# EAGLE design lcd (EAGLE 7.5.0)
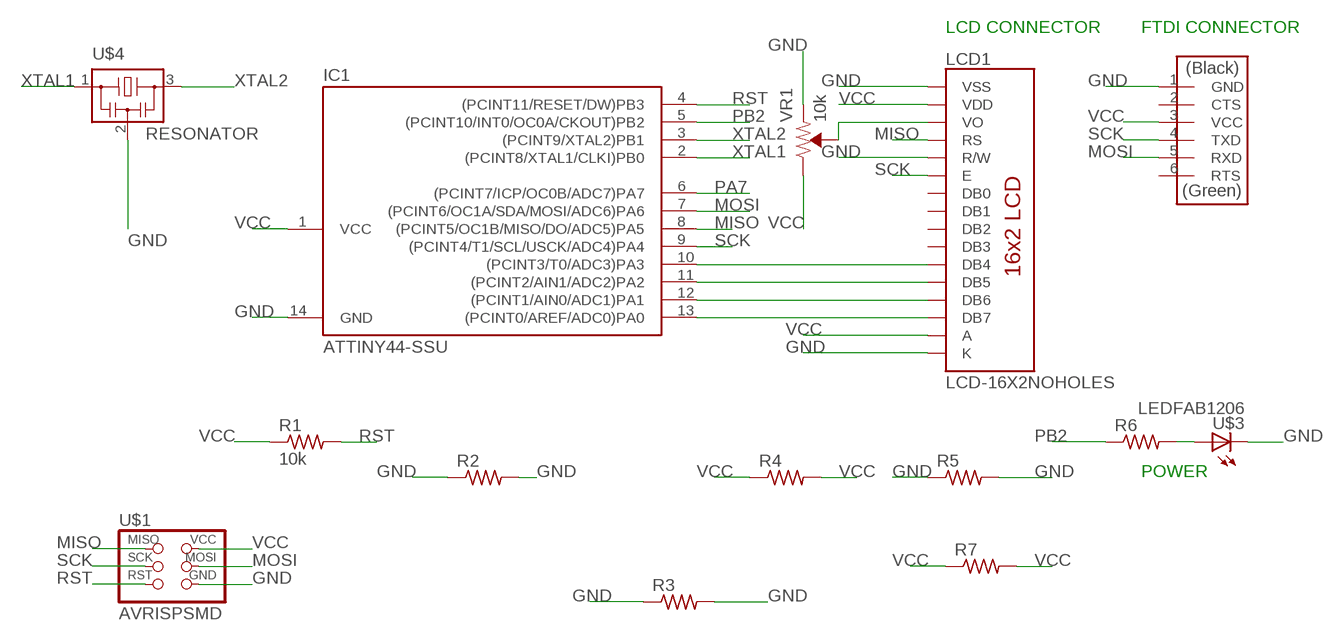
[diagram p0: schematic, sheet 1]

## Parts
IC1  ATTINY44-SSU  [SOIC14]
LCD1  LCD-16X2NOHOLES  [LCD-16X2_NOHOLESNOSILK]
R1  10k  RES-US1206FAB  [R1206FAB]
R2  RES-US1206FAB  [R1206FAB]
R3  RES-US1206FAB  [R1206FAB]
R4  RES-US1206FAB  [R1206FAB]
R5  RES-US1206FAB  [R1206FAB]
R6  RES-US1206FAB  [R1206FAB]
R7  RES-US1206FAB  [R1206FAB]
U$1  AVRISPSMD  [2X03SMD]
U$2  FTDI-SMD-HEADER  [1X06SMD]
U$3  LEDFAB1206  [LED1206FAB]
U$4  RESONATOR  [EFOBM]
VR1  10k  TRIMPOT-PTH-10MM-KNOB-1/2W-10%  [TRIMPOT-PTH-3386U]

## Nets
GND: IC1.14(GND) LCD1.1(VSS) LCD1.5(R/W) LCD1.16(K) R2.1 R2.2 R3.1 R3.2 R5.1 R5.2 U$1.6(GND) U$2.1(GND) U$3.2(C) U$4.2 VR1.1(CCW)
MISO: IC1.8((PCINT5/OC1B/MISO/DO/ADC5)PA5) LCD1.4(RS) U$1.1(MISO)
MOSI: IC1.7((PCINT6/OC1A/SDA/MOSI/ADC6)PA6) U$1.4(MOSI) U$2.5(RXD)
N$1: R6.2 U$3.1(A)
N$2: LCD1.3(VO) VR1.2(WIPER)
N$3: IC1.10((PCINT3/T0/ADC3)PA3) LCD1.11(DB4)
N$4: IC1.11((PCINT2/AIN1/ADC2)PA2) LCD1.12(DB5)
N$5: IC1.12((PCINT1/AIN0/ADC1)PA1) LCD1.13(DB6)
N$6: IC1.13((PCINT0/AREF/ADC0)PA0) LCD1.14(DB7)
PA7: IC1.6((PCINT7/ICP/OC0B/ADC7)PA7)
PB2: IC1.5((PCINT10/INT0/OC0A/CKOUT)PB2) R6.1
RST: IC1.4((PCINT11/RESET/DW)PB3) R1.2 U$1.5(RST)
SCK: IC1.9((PCINT4/T1/SCL/USCK/ADC4)PA4) LCD1.6(E) U$1.3(SCK) U$2.4(TXD)
VCC: IC1.1(VCC) LCD1.2(VDD) LCD1.15(A) R1.1 R4.1 R4.2 R7.1 R7.2 U$1.2(VCC) U$2.3(VCC) VR1.3(CW)
XTAL1: IC1.2((PCINT8/XTAL1/CLKI)PB0) U$4.1
XTAL2: IC1.3((PCINT9/XTAL2)PB1) U$4.3
Unconnected: LCD1.7(DB0) LCD1.8(DB1) LCD1.9(DB2) LCD1.10(DB3) U$2.2(CTS) U$2.6(RTS)

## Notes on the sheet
- LCD CONNECTOR | FTDI CONNECTOR
- POWER

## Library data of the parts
IC1 = fab:ATTINY44
LCD1 = SparkFun-Displays:LCD-16X2: Standard text-only 16x2 parallel input LCD Basic 16 character by 2 line display. Typically utilizes the extremely common HD44780 parallel interface chipset SparkFun Products: Basic 16x2 Green Basic 8x2 Green; SF_ID: LCD-00255
R1-R7 = fab:RES-US: Resistor (US Symbol)
U$1 = fab:AVRISP
U$2 = fab:FTDI-SMD-HEADER
U$3 = fab:LED: LED
U$4 = fab:RESONATOR
VR1 = SparkFun-Resistors:TRIMPOT: Trimming Potentiometer (Trimpot) Three-terminal potentiometers, with an adjustable wiper and two adjustable resistors. A pot can be used to create a configurable voltage divider, or as a variable resistor. "Trimpots" are a subset of potentiometers, usually intended for "set-and-forget"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; PROD_ID: RES-09730; SF_SKU: COM-09806

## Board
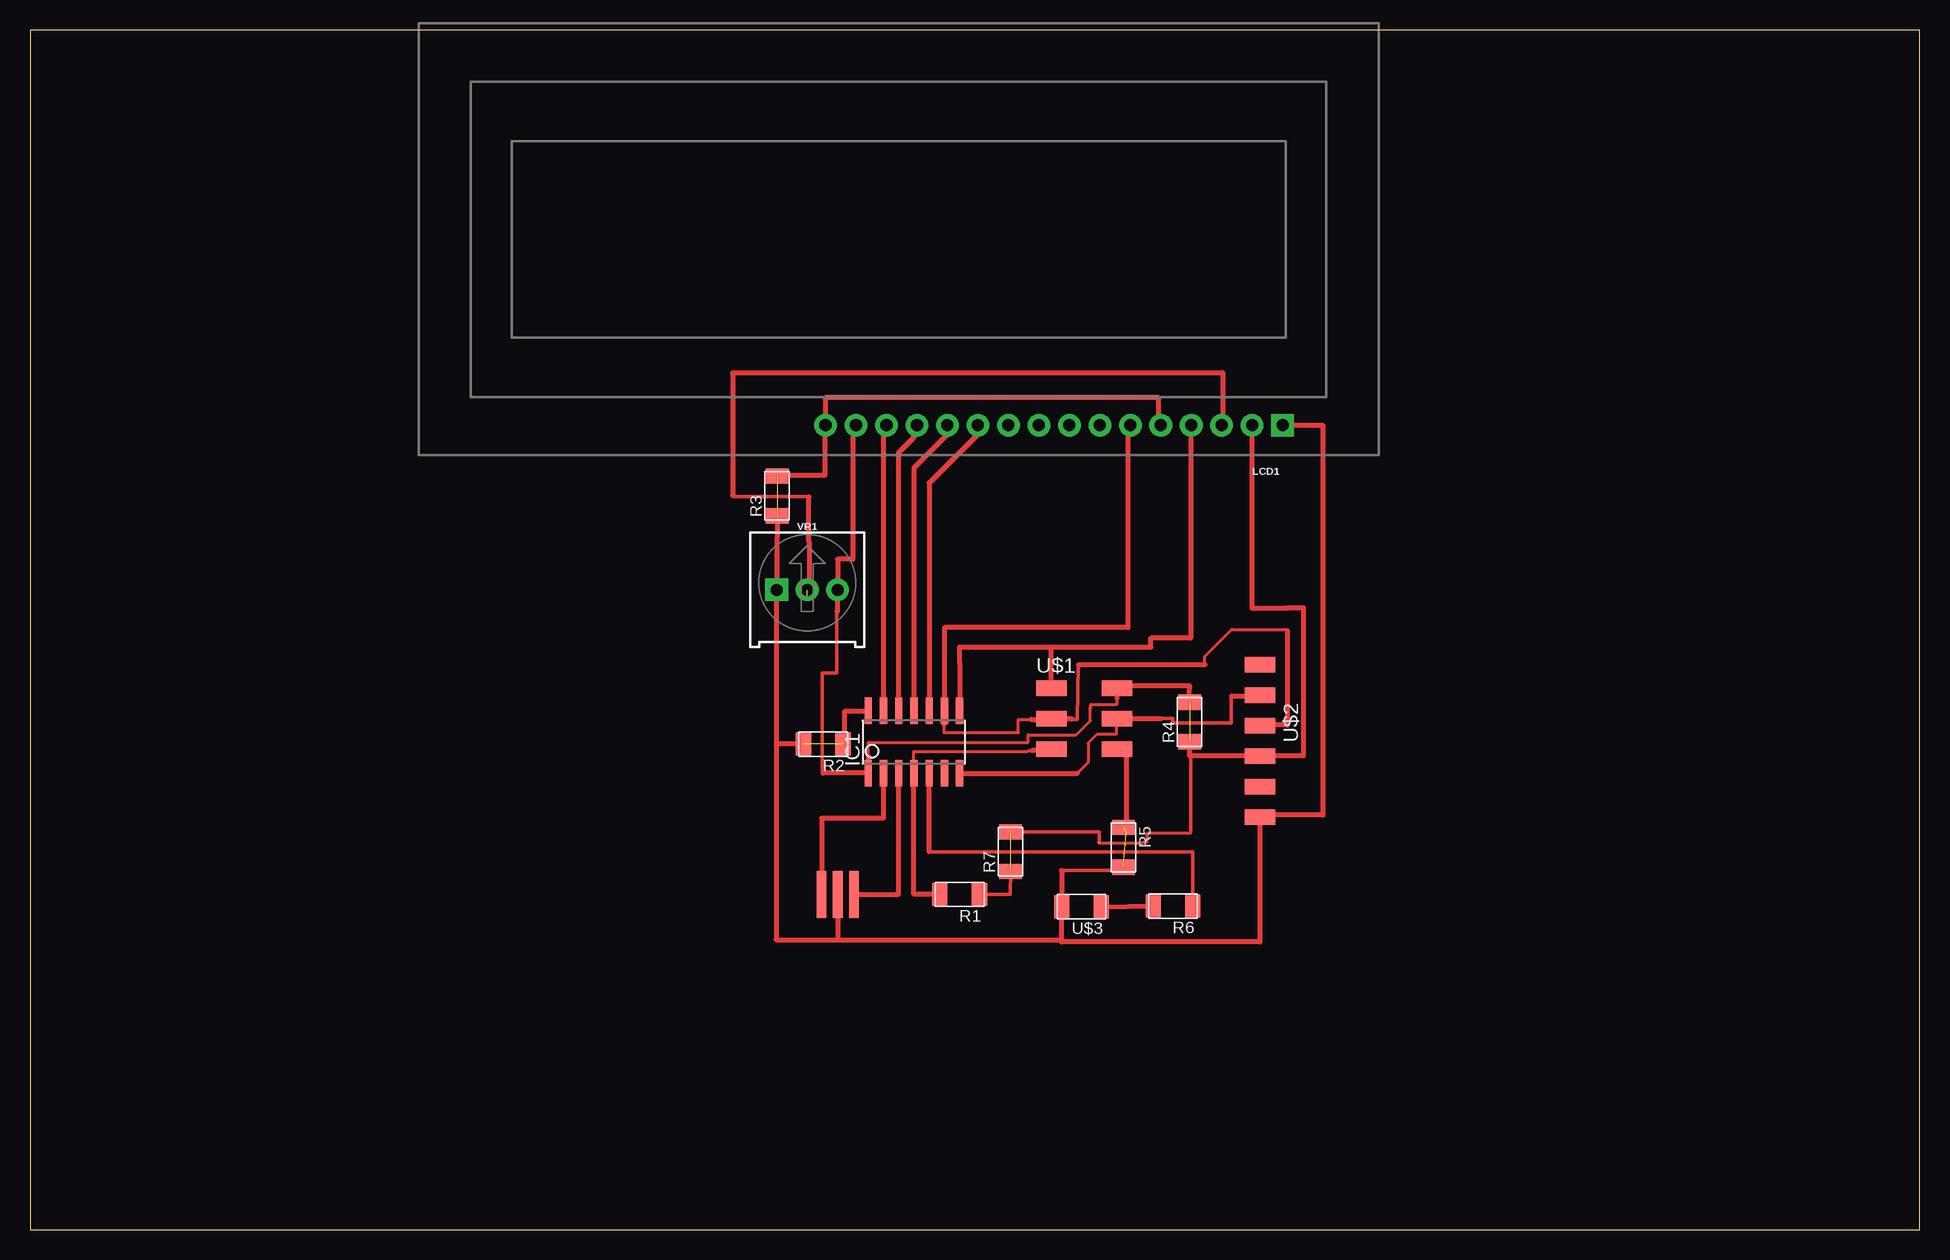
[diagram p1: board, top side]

Size 157.46 x 100 mm. Coordinates in mm from the lower left corner, seen from the top.
Outline: 0,0 157.46,0 157.46,100 0,100 0,0
Copper layers (1*16): Top 0.035mm / dielectric 1.5mm / Bottom 0.035mm
Design rules "default": minimum track width 10mil, minimum drill 24mil, track to track 8mil, track to pad 8mil, pad to pad 8mil, via to via 8mil, smd to smd 8mil, copper to edge 40mil, drill to drill 8mil, minimum pad ring 10mil, minimum via ring 8mil, stop-mask expansion 4mil, vias tented up to drill 0mil, thermal gap 10mil

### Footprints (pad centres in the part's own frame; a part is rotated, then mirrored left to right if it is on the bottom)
SOIC14 = smd 0.61 x 2.21: 1 -3.81,-2.603; 2 -2.54,-2.603; 3 -1.27,-2.603; 4 0,-2.603; 5 1.27,-2.603; 6 2.54,-2.603; 7 3.81,-2.603; 8 3.81,2.603; 9 2.54,2.603; 10 1.27,2.603; 11 0,2.603; 12 -1.27,2.603; 13 -2.54,2.603; 14 -3.81,2.603
LCD-16X2_NOHOLESNOSILK = drill 1.016 pad 1.88 square: 1 -32,15.5 | drill 1.016 pad 1.88: 2 -29.46,15.5; 3 -26.92,15.5; 4 -24.38,15.5; 5 -21.84,15.5; 6 -19.3,15.5; 7 -16.76,15.5; 8 -14.22,15.5; 9 -11.68,15.5; 10 -9.14,15.5; 11 -6.6,15.5; 12 -4.06,15.5; 13 -1.52,15.5; 14 1.02,15.5; 15 3.56,15.5; 16 6.1,15.5
R1206FAB = smd 1.27 x 1.905: 1 -1.651,0; 2 1.651,0
2X03SMD = smd 2.54 x 1.27: 1 -2.54,2.54; 2 2.92,2.54; 3 -2.54,0; 4 2.92,0; 5 -2.54,-2.54; 6 2.92,-2.54
1X06SMD = smd 2.54 x 1.27: 1 0,6.35; 2 0,3.81; 3 0,1.27; 4 0,-1.27; 5 0,-3.81; 6 0,-6.35
LED1206FAB = smd 1.27 x 1.905: 1 -1.651,0; 2 1.651,0
EFOBM = smd 0.8 x 3.9: 1 -1.35,0; 2 0,0; 3 1.35,0
TRIMPOT-PTH-3386U = drill 1.016 pad 1.88 square: 1 -2.54,-0.015 | drill 1.016 pad 1.88: 2 0,-0.015; 3 2.54,-0.015

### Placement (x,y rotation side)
IC1  73.66,40.64 0 top
LCD1  72.39,82.55 180 top
R1  77.47,27.94 180 top
R2  66.1,40.47 180 top
R3  62.26,61.16 90 top
R4  96.64,42.32 90 top
R5  91.12,31.86 270 top
R6  95.25,26.97 180 top
R7  81.71,31.5 90 top
U$1  87.66,42.59 0 top
U$2  102.52,40.73 180 top
U$3  87.63,26.91 180 top
U$4  67.31,27.94 0 top
VR1  64.77,53.34 0 top

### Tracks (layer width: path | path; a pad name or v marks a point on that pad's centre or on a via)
GND  (4 unrouted)
  Top 0.305: 85.98,29.93 91.12,29.93 R5.2
  Top 0.406: U$4.2 67.31,24.16 | 85.98,24.13 67.31,24.13 67.31,24.16 | 85.98,24.13 U$3.2 85.98,29.93 | 85.98,24.13 85.98,23.97 102.52,23.97 U$2.1 102.52,34.56 107.74,34.56 107.74,67.05 LCD1.1 | 62.18,40.47 62.18,53.33 VR1.1 62.23,55.91 R3.1 | 62.18,40.47 62.18,24.16 67.31,24.16 | 69.68,43.24 IC1.14 69.85,43.22 67.9,43.22 67.9,40.5 67.75,40.5 R2.1 | R2.2 62.18,40.47 | 66.29,67.38 LCD1.16 | LCD1.5 94.05,67.05 94.05,69.34 66.29,69.34 LCD1.16 | U$1.6 91.33,40.05 91.33,33.06 | LCD1.16 66.24,67.05 66.24,62.88 62.26,62.88 R3.2
MISO
  Top 0.406: IC1.8 77.47,47.28 77.46,47.28 77.46,48.56 85.08,48.56 | U$1.1 85.08,45.12 | LCD1.4 96.71,67.05 96.71,49.31 93.4,49.31 93.4,48.56 85.08,48.56 | 85.02,45.12 85.08,45.12 | 85.08,45.12 85.08,48.56
MOSI
  Top 0.254: U$1.4 90.55,41.28 88.9,41.28 88.18,40.56 88.18,38.94 87.27,38.04
  Top 0.305: 94.24,42.59 95.21,42.59 95.21,42.25 100.12,42.25 100.12,44.47
  Top 0.406: 90.58,42.53 U$1.4 94.24,42.59 | 77.47,37.97 IC1.7 87.27,38.04 | 100.12,44.47 102.52,44.47 U$2.5
N$1
  Top 0.406: U$3.1 R6.2
N$2  (1 unrouted)
  Top 0.305: 64.9,61.09 58.55,61.09 58.55,61.22
  Top 0.406: LCD1.3 99.43,67.05 99.43,71.41 58.55,71.41 58.55,61.22 | 64.77,52.78 64.93,52.78 64.93,57.34 64.9,57.34 64.9,61.09
N$3
  Top 0.406: LCD1.11 78.99,66.29 74.93,62.23 IC1.10
N$4
  Top 0.406: LCD1.12 76.45,66.29 73.66,63.5 IC1.11
N$5
  Top 0.406: IC1.12 72.39,64.77 73.66,66.04 73.66,66.8 LCD1.13
N$6
  Top 0.406: LCD1.14 71.12,67.05 IC1.13
PB2
  Top 0.305: 74.93,31.5 96.9,31.5 R6.1
  Top 0.406: 96.71,26.97 R6.1 96.99,26.97 | 74.93,31.5 IC1.5
RST
  Top 0.254: 73.62,39.06 73.65,39.06 73.65,39.88 83.15,39.88 83.15,39.94 83.49,39.94
  Top 0.406: R1.2 73.66,27.94 IC1.4 73.62,38.04 73.62,39.06 | U$1.5 84.68,40.05 84.68,39.94 83.49,39.94
SCK
  Top 0.254: 76.18,42.09 76.15,42.09 76.15,41.44 82.37,41.44 82.37,42.53 83.4,42.53 | 97.9,47.09 97.9,47.78 100.15,50.03 104.65,50.03 104.77,49.91
  Top 0.305: 86.8,42.53 87.27,42.53 87.37,47.09
  Top 0.406: IC1.9 76.18,43.24 76.18,42.09 | 76.24,43.24 IC1.9 | IC1.9 76.21,50.19 91.49,50.19 91.49,67.05 LCD1.6 | 87.37,47.09 97.9,47.09 | 104.77,49.91 104.77,42.06 102.52,42.06 U$2.4 | 83.4,42.53 85.12,42.53 U$1.3 86.8,42.59 86.8,42.53
VCC  (3 unrouted)
  Top 0.254: 69.9,39.44 69.87,39.44 69.87,40.62 83.18,40.62 83.18,41.25 87.18,41.25 88.37,42.41 88.37,43.5 88.43,43.78 90.55,43.78 90.58,43.81 90.58,44.28 | 89.02,32.25 92.74,32.25 92.74,32.31 93.08,32.31 93.08,33.06 96.71,33.06 96.71,33.16
  Top 0.305: 66.08,38.12 66.02,38.12 66.02,46.41 67.24,46.41 67.24,51.56 | R1.1 81.68,27.94 R7.1 | 96.71,33.16 96.71,39.5 | 89.08,32.25 89.08,33.16 R7.2
  Top 0.406: LCD1.15 68.58,67.05 68.58,55.88 67.31,55.88 VR1.3 67.31,51.56 67.24,51.56 | U$2.3 101.95,39.5 | LCD1.2 101.85,51.81 104.83,51.81 104.83,51.84 106.12,51.84 106.12,39.5 101.95,39.5 | 90.58,44.28 U$1.2 90.68,45.31 96.65,45.31 96.55,43.97 R4.2 | 69.9,39.44 69.9,38.04 IC1.1 69.85,38.06 66.08,38.06 66.08,38.12 | 101.95,39.5 96.71,39.5 96.64,39.5 R4.1
XTAL1
  Top 0.406: IC1.2 71.12,34.29 65.96,34.29 U$4.1
XTAL2
  Top 0.406: U$4.3 72.39,27.94 IC1.3 72.39,38.1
